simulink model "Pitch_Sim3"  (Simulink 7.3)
settings: Solver=ode45  StartTime=0.0  StopTime=200  RelTol=1e-3
InitFcn:
  | init
StartFcn:
  | init
StopFcn:
  | pl
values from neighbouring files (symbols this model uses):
  Cza = -0.032    [init.m]    (also in init_pitch.m)
  Czde = -0.0087    [init.m]    (also in init_pitch.m)
  d2r = 1/r2d    (= 0.0174532925199)    [init.m]    (also in freq.m; frequ.m; init_lat.m; pl.m)
  Mv = 1219.1    [init.m]    (also in init_lat.m; init_pitch.m)
  Qbar = 1220.6    [init.m]    (also in init_lat.m; init_pitch.m)
  r2d = 180/pi    (= 57.2957795131)    [init.m]    (also in freq.m; frequ.m; init_lat.m; pl.m)
  Sref = 145.4    [init.m]    (also in init_lat.m; init_pitch.m)
undefined symbols (not defined in the file or in its folder): Ap, Bp, Cp, Dp

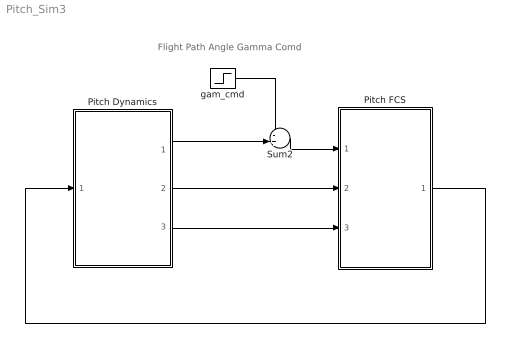
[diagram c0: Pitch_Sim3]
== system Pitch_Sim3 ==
  note: Flight Path Angle Gamma Comd
  Pitch Dynamics : Subsystem
  Pitch FCS : Subsystem
  Sum2 : Sum  Inputs=-+|  OutDataType=fixdt(1, 16)  OutScaling=2^0
  gam_cmd : Step  After=d2r  SampleTime=0
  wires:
  Pitch Dynamics/2(q) -> Pitch FCS/2(q)
  Pitch Dynamics/3(Nz) -> Pitch FCS/3(Nz)
  Pitch Dynamics/1(gamma) -> Sum2/2
  Sum2/1 -> Pitch FCS/1(gamerr)
  Pitch FCS/1(d-elev) -> Pitch Dynamics/1(elev)
  gam_cmd/1 -> Sum2/1

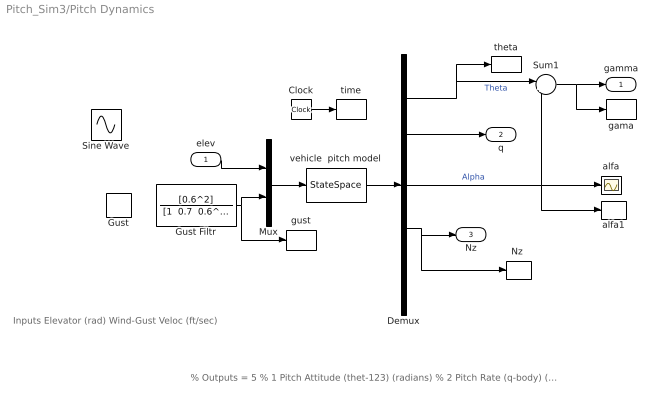
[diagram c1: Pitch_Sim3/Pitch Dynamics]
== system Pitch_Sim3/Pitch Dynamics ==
  note: % Outputs = 5 % 1 Pitch Attitude (thet-123) (radians) % 2 Pitch Rate (q-body) (rad/sec) % 3 Angle of attack, alfa, (radians) % 4 Accelerom # 2, (along Z), (ft/sec^2) Translat. Acceler % 5 Alpha Sensed at Vane # 1 (radian)
  note: Inputs Elevator (rad) Wind-Gust Veloc (ft/sec)
  elev : Inport
  Clock : Clock
  Demux : Demux  Outputs=5
  Gust : DiscretePulseGenerator  PulseType=Time based  Amplitude=30  Period=500  PulseWidth=2  PhaseDelay=0  SampleTime=1
  Gust Filtr : TransferFcn  Numerator=[0.6^2]  Denominator="[1  0.7  0.6^2]"
  Mux : Mux  Inputs=2
  "Nz " : ToWorkspace  VariableName=Nz  SampleTime=-1  SaveFormat=Array
  Sine Wave : Sin  Amplitude=30  Bias=0  Frequency=0.3  Phase=0  Samples=10  SampleTime=0
  Sum1 : Sum  Inputs=|+-  OutDataType=fixdt(1, 16)  OutScaling=2^0
  alfa : Scope
  alfa1 : ToWorkspace  VariableName=alfa  SampleTime=-1  SaveFormat=Array
  gama : ToWorkspace  VariableName=gama  SampleTime=-1  SaveFormat=Array
  gust : ToWorkspace  VariableName=Vgst  SampleTime=-1  SaveFormat=Array
  theta : ToWorkspace  VariableName=theta  SampleTime=-1  SaveFormat=Array
  time : ToWorkspace  VariableName=time  SampleTime=-1  SaveFormat=Array
  vehicle  pitch model : StateSpace  A=Ap  B=Bp  C=Cp  D=Dp
  gamma : Outport
  q : Outport  Port=2
  Nz : Outport  Port=3
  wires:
  vehicle  pitch model/1 -> Demux/1
  Mux/1 -> vehicle  pitch model/1
  Demux/2 -> q/1
  elev/1 -> Mux/1
  Demux/3 -> Sum1/2, alfa/1, alfa1/1  "Alpha"
  Demux/4 -> Nz/1, "Nz "/1
  Sum1/1 -> gamma/1, gama/1
  Demux/1 -> Sum1/1, theta/1  "Theta"
  Gust Filtr/1 -> Mux/2, gust/1
  Clock/1 -> time/1

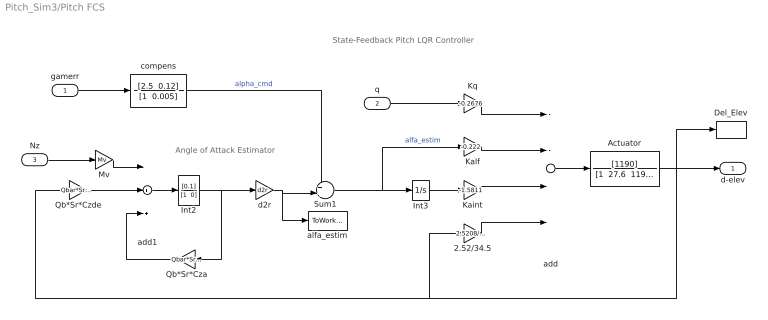
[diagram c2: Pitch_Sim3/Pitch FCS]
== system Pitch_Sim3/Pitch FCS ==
  note: Angle of Attack Estimator
  note: State-Feedback Pitch LQR Controller
  gamerr : Inport
  q : Inport  Port=2
  Nz : Inport  Port=3
  2.52/34.5 : Gain  Gain=2.5208/34.5  ParameterDataType=fixdt(1, 16)  ParameterScaling=2^0  OutDataType=fixdt(1, 16)  OutScaling=2^0
  Actuator : TransferFcn  Numerator=[1190]  Denominator="[1  27.6  1190]"
  Del_Elev : ToWorkspace  VariableName=delev  SampleTime=-1  SaveFormat=Array
  Int2 : TransferFcn  Numerator=[0.1]  Denominator="[1  0]"
  Int3 : Integrator
  Kaint : Gain  Gain=-1.5811  ParameterDataType=fixdt(1, 16)  ParameterScaling=2^0  OutDataType=fixdt(1, 16)  OutScaling=2^0
  Kalf : Gain  Gain=-0.222  ParameterDataType=fixdt(1, 16)  ParameterScaling=2^0  OutDataType=fixdt(1, 16)  OutScaling=2^0
  Kq : Gain  Gain=-0.2676  ParameterDataType=fixdt(1, 16)  ParameterScaling=2^0  OutDataType=fixdt(1, 16)  OutScaling=2^0
  Mv : Gain  Gain=Mv  ParameterDataType=fixdt(1, 16)  ParameterScaling=2^0  OutDataType=fixdt(1, 16)  OutScaling=2^0
  Qb*Sr*Cza : Gain  Gain=Qbar*Sref*Cza  ParameterDataType=fixdt(1, 16)  ParameterScaling=2^0  OutDataType=fixdt(1, 16)  OutScaling=2^0
  Qb*Sr*Czde : Gain  Gain=Qbar*Sref*Czde*r2d  ParameterDataType=fixdt(1, 16)  ParameterScaling=2^0  OutDataType=fixdt(1, 16)  OutScaling=2^0
  Sum1 : Sum  Inputs=++|  OutDataType=fixdt(1, 16)  OutScaling=2^0
  add : Sum  Inputs=----  OutDataType=fixdt(1, 16)  OutScaling=2^-10
  add1 : Sum  Inputs=-++  OutDataType=fixdt(1, 16)  OutScaling=2^-10
  alfa_estim : ToWorkspace  VariableName=alfa_est  SampleTime=-1  SaveFormat=Array
  compens : TransferFcn  Numerator="[2.5  0.12]"  Denominator="[1  0.005]"
  d2r : Gain  Gain=d2r  ParameterDataType=fixdt(1, 16)  ParameterScaling=2^0  OutDataType=fixdt(1, 16)  OutScaling=2^0
  d-elev : Outport
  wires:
  d2r/1 -> Sum1/2, alfa_estim/1
  Nz/1 -> Mv/1
  Int2/1 -> Qb*Sr*Cza/1, d2r/1
  Qb*Sr*Czde/1 -> add1/2
  Mv/1 -> add1/1
  Qb*Sr*Cza/1 -> add1/3
  add1/1 -> Int2/1
  gamerr/1 -> compens/1
  compens/1 -> Sum1/1  "alpha_cmd"
  Actuator/1 -> Qb*Sr*Czde/1, 2.52/34.5/1, d-elev/1, Del_Elev/1
  add/1 -> Actuator/1
  q/1 -> Kq/1
  2.52/34.5/1 -> add/4
  Kaint/1 -> add/3
  Int3/1 -> Kaint/1
  Sum1/1 -> Int3/1, Kalf/1  "alfa_estim"
  Kq/1 -> add/1
  Kalf/1 -> add/2
